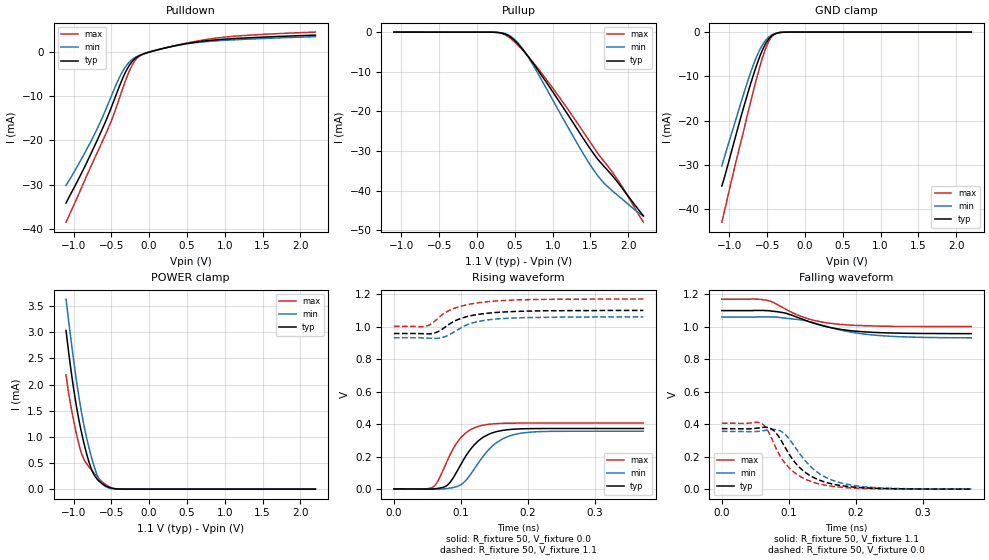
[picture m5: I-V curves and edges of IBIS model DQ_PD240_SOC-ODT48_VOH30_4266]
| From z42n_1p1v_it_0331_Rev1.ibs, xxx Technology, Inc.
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| DQ_PD240_SOC-ODT48_VOH30_4266
| (240 Ohm Pulldown, 48 Ohm System ODT Setting, VOH=VDDQ/3.0, 3200-4266Mbps)
[Model]   DQ_PD240_SOC-ODT48_VOH30_4266
Model_type   I/O
Vinl = 123.333mV
Vinh = 243.333mV
Vmeas = 183.333mV
Vref = 0.0mV
Cref = 0.0pF
Rref = 48.000Ohm
|   typ   min   max
|C_comp   0.834pF   0.784pF   0.884pF
C_comp_pullup   0.4170pF   0.3920pF   0.4420pF
C_comp_pulldown   0.4170pF   0.3920pF   0.4420pF
| Note: C_comp changes when the ODT circuit is enabled.
[Model Spec]
| Input threshold voltage corners
Vinl   0.1233V   0.1167V   0.1350V
Vinh   0.2433V   0.2367V   0.2550V
| Measurement voltage corners
Vmeas   0.1833V   0.1767V   0.1950V
| Timing spec test load voltage corners
Vref   0.0000V   0.0000V   0.0000V
| Dynamic Overshoot Parameters from LPDDR4 Specification
D_overshoot_ampl_h   0.30   NA   NA
D_overshoot_ampl_l   0.30   NA   NA
D_overshoot_area_h   0.1n   NA   NA
D_overshoot_area_l   0.1n   NA   NA
[Voltage Range]   1.1000V   1.0600V   1.1700V
[Pullup Reference]   1.1000V   1.0600V   1.1700V
| Junction Temperature (Ambient temp is 35C typ 95C min -40C max)
[Temperature Range]   50.0   110.0   -40.0
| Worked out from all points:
|   slope of the pulldown table from 0 to 0.165 V, typ, clamps not added: 222 ohm
|   slope of the pullup table from 0 to 0.165 V, typ, clamps not added: 15.7 kohm
|   GND clamp passes 1 mA (typ) near -0.45 V on its own axis
|   POWER clamp passes 1 mA (typ) near -0.88 V on its own axis
|   rising waveform, R_fixture 50, V_fixture 0.0: 20-80 % time 37.1ps typ, 41.9ps min, 32.4ps max; typ from 0.001 V to 0.373 V
|   falling waveform, R_fixture 50, V_fixture 1.1: 20-80 % time 69.5ps typ, 80.6ps min, 59.2ps max; typ from 1.1 V to 0.958 V
|   rising waveform, R_fixture 50, V_fixture 1.1: 20-80 % time 46.9ps typ, 43.9ps min, 49ps max; typ from 0.958 V to 1.1 V
|   falling waveform, R_fixture 50, V_fixture 0.0: 20-80 % time 46.6ps typ, 50.8ps min, 42.7ps max; typ from 0.373 V to 0.001 V
[Pulldown]
|   Voltage   I(typ)   I(min)   I(max)
-1.1V     -34.14mA   -30.13mA   -38.47mA
-925.1mV  -28.42mA   -25.08mA   -31.88mA
-720.5mV  -21.19mA   -18.51mA   -24.01mA
-499.4mV  -12.48mA   -9.914mA   -15.51mA
-357.5mV  -6.246mA   -4.591mA   -8.628mA
-291.5mV  -3.863mA   -2.855mA   -5.528mA
-232.1mV  -2.3mA     -1.803mA   -3.23mA
-133.1mV  -878.4uA   -794.1uA   -994.8uA
-17.6mV   -114uA     -109.1uA   -105.8uA
338.8mV   1.399mA    1.377mA    1.431mA
807.4mV   2.621mA    2.422mA    2.952mA
2.2V      3.814mA    3.471mA    4.502mA
[GND Clamp]
|   Voltage   I(typ)   I(min)   I(max)
-1.1V     -34.74mA   -30.21mA   -42.91mA
-1.05V    -31.86mA   -27.33mA   -39.27mA
-944.9mV  -25.23mA   -21.44mA   -31.55mA
-793.1mV  -15.92mA   -12.96mA   -20.95mA
-667.7mV  -8.907mA   -6.722mA   -12.29mA
-591.8mV  -5.255mA   -3.789mA   -7.492mA
-525.8mV  -2.766mA   -1.974mA   -3.964mA
-473mV    -1.425mA   -1.032mA   -1.887mA
-416.9mV  -600.2uA   -440.5uA   -664.9uA
-350.9mV  -166.8uA   -126.3uA   -148.2uA
-248.6mV  -12.31uA   -11.02uA   -7.125uA
2.2V      0A         0A         0A
[Pullup]
|   Voltage   I(typ)   I(min)   I(max)
-1.1V     5.229uA    8.059uA    2.358uA
233.2mV   -40.35uA   -40.62uA   -42.13uA
335.5mV   -286.4uA   -235.7uA   -391.6uA
431.2mV   -1.117mA   -909.9uA   -1.417mA
550mV     -3.186mA   -2.926mA   -3.464mA
682mV     -6.308mA   -6.472mA   -6.26mA
1.091V    -17.65mA   -20.22mA   -16.5mA
1.391V    -26.44mA   -30.26mA   -24.79mA
1.566V    -31.33mA   -35.46mA   -29.76mA
1.675V    -33.81mA   -38.02mA   -32.54mA
1.867V    -38.07mA   -41.32mA   -37.5mA
2.2V      -46.44mA   -46.37mA   -47.99mA
[POWER Clamp]
|   Voltage   I(typ)   I(min)   I(max)
-1.1V     3.033mA    3.633mA    2.184mA
-1.044V   2.381mA    2.967mA    1.653mA
-977.9mV  1.723mA    2.241mA    1.16mA
-908.6mV  1.177mA    1.583mA    748uA
-852.5mV  818.4uA    1.149mA    543.5uA
-776.6mV  434.1uA    683.2uA    390.2uA
-713.9mV  239.2uA    373uA      278.6uA
-661.1mV  151.1uA    187.5uA    195.4uA
-598.4mV  83.65uA    72.01uA    113uA
-492.8mV  18.96uA    11.63uA    24.05uA
-383.9mV  1.761uA    1.219uA    1.465uA
2.2V      0A         0A         0A
[Ramp]
|   typ   min   max
| 20% - 80%
dV/dt_r   223.43m/37.14p   213.40m/41.93p   243.75m/32.37p
dV/dt_f   85.15m/69.43p   76.64m/80.24p   100.80m/58.91p
| 25% - 75%
|dV/dt_r   186.19m/29.60p   177.83m/33.34p   203.13m/25.80p
|dV/dt_f   70.96m/55.26p   63.87m/63.47p   84.00m/46.80p
R_load = 50
[Rising Waveform]
R_fixture = 50
V_fixture = 0.0
|   Time   V(typ)   V(min)   V(max)
0s        944.6uV    840.9uV    678.4uV
57ps      597.9uV    -79.9uV    9.862mV
65ps      3.879mV    -354.8uV   45.63mV
77ps      16.92mV    2.586mV    151.7mV
86ps      54.38mV    7.944mV    230.4mV
100ps     153.3mV    27.31mV    317.4mV
128ps     304mV      173.5mV    388.7mV
154ps     354.9mV    288.7mV    403.5mV
186ps     370.4mV    341.7mV    406.6mV
372ps     373.3mV    356.5mV    406.9mV
[Falling Waveform]
R_fixture   = 50
V_fixture   = 1.1
V_fixture_min = 1.06
V_fixture_max = 1.17
|   Time   V(typ)   V(min)   V(max)
0s        1.1V       1.06V      1.17V
50ps      1.101V     1.06V      1.171V
69ps      1.099V     1.061V     1.162V
97ps      1.082V     1.052V     1.105V
123ps     1.043V     1.039V     1.057V
140ps     1.019V     1.021V     1.037V
168ps     990.7mV    989.1mV    1.018V
203ps     972.1mV    960.7mV    1.008V
242ps     963.2mV    944.3mV    1.004V
372ps     958.1mV    932.3mV    1.002V
[Rising Waveform]
R_fixture   = 50
V_fixture   = 1.1
V_fixture_min = 1.06
V_fixture_max = 1.17
|   Time   V(typ)   V(min)   V(max)
0s        957.9mV    931.6mV    1.002V
45ps      956mV      930.6mV    1.001V
56ps      956.9mV    928mV      1.018V
70ps      979.2mV    930.9mV    1.067V
81ps      1.011V     947.2mV    1.097V
96ps      1.045V     984.1mV    1.121V
113ps     1.066V     1.018V     1.138V
132ps     1.079V     1.037V     1.151V
204ps     1.096V     1.057V     1.167V
372ps     1.1V       1.06V      1.17V
[Falling Waveform]
R_fixture = 50
V_fixture = 0.0
|   Time   V(typ)   V(min)   V(max)
0s        373.4mV    356.7mV    407mV
56ps      378.7mV    357.3mV    410.2mV
73ps      374.3mV    367.6mV    324.8mV
86ps      317.1mV    361.9mV    210.8mV
100ps     218.5mV    311.8mV    133.7mV
118ps     125.9mV    208.4mV    76.18mV
140ps     66mV       112.3mV    38.75mV
167ps     30.57mV    52.38mV    17.18mV
204ps     11.13mV    19.29mV    5.941mV
372ps     1.102mV    1.123mV    726.4uV
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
